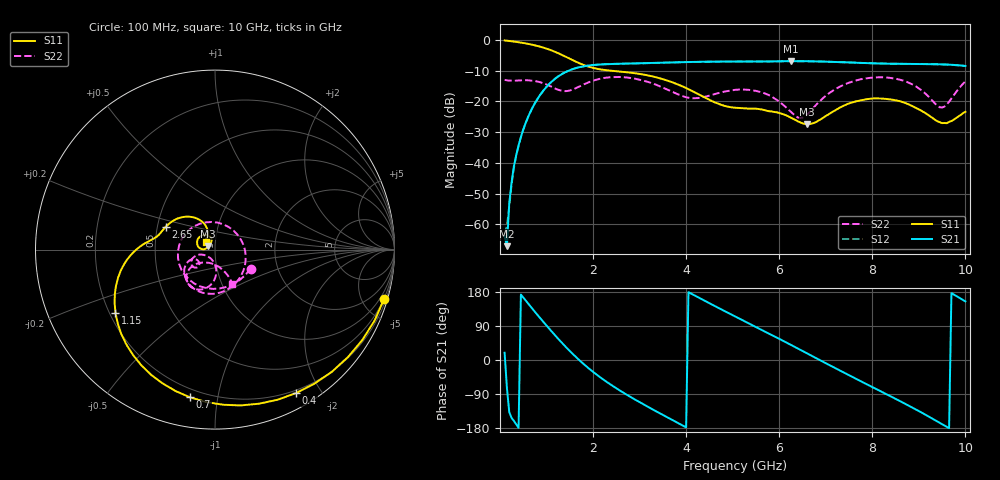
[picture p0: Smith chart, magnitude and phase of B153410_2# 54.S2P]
!  2-Port S-parameters saved by WinCal
! VAR MeasName=S-Parameters (CALIBRATED_DATA) read from VNA (N5245A)
! VAR MeasDate=2016-12-23 10:02:13
! VAR NAME=B153410_2# 54
! VAR FILENAME=B153410_2# 54.S2P
! VAR DATE=2016-12-23 10:02:13
! VAR PHYS_PORTS=1,2
# Hz S DB R 50
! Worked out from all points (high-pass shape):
!   199 points, 100 MHz to 10 GHz, reference 50 ohm
!   highest |S21| = -6.89 dB at 6.25 GHz (marker M1); lowest = -67.1 dB at 150 MHz (marker M2)
!   |S21| within 3 dB of the highest: 1.491 GHz to end of sweep
!   lowest |S11| = -27.4 dB at 6.6 GHz (marker M3), VSWR 1.09, Z = 46.3 + j1.88 ohm
!   |S11| at or under -10 dB: 2.386 GHz to end of sweep
!   |S22| runs from -25.4 to -12.0 dB; largest |S21 - S12| = 0.0019
!   S11 on the Smith chart (normalised r, x): 100 MHz: 0.46, -7.02; 400 MHz: 0.17, -1.70; 700 MHz: 0.15, -0.83; 1.15 GHz: 0.22, -0.28; 2.65 GHz: 0.55, +0.15; 10 GHz: 0.90, +0.08
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1e8  -0.16 -16.2  -63.69 19.3  -63.06 34.0  -12.97 -28.1
1.5e8  -0.24 -23.9  -67.07 -74.4  -60.59 -79.3  -13.12 -39.8
2e8  -0.33 -31.5  -53.02 -137.7  -54.10 -133.6  -13.22 -51.0
2.5e8  -0.42 -38.9  -46.35 -152.7  -46.99 -147.7  -13.22 -62.1
4e8  -0.74 -60.5  -34.27 -178.9  -34.47 -179.1  -13.18 -92.7
7e8  -1.57 -99.6  -22.00 134.8  -21.97 135.0  -13.23 -148.7
1.15e9  -3.65 -147.5  -13.05 69.9  -13.01 69.8  -15.52 121.1
1.75e9  -7.85 176.3  -8.72 -5.4  -8.70 -5.5  -14.83 -20.2
2.2e9  -9.67 166.5  -7.94 -49.7  -7.93 -49.8  -12.46 -79.5
2.65e9  -10.38 155.3  -7.72 -86.2  -7.72 -86.2  -12.11 -116.8
3.4e9  -12.32 130.7  -7.45 -138.4  -7.45 -138.5  -14.85 -153.1
4.2e9  -17.16 111.1  -7.13 169.2  -7.14 169.2  -18.95 -143.4
5.05e9  -22.04 126.0  -7.02 114.9  -7.04 115.0  -16.23 -140.5
5.7e9  -22.89 130.9  -7.00 74.4  -7.01 74.5  -17.44 -158.5
6.25e9  -25.30 132.6  -6.89 40.0  -6.92 39.9  -23.39 -153.7
6.6e9  -27.40 151.6  -6.91 17.4  -6.93 17.4  -24.26 -103.7
6.7e9  -27.23 159.9  -6.94 11.0  -6.96 10.9  -22.66 -94.3
7.4e9  -21.28 174.3  -7.26 -33.8  -7.26 -33.9  -14.49 -94.8
8.35e9  -19.27 135.8  -7.72 -93.1  -7.72 -93.0  -12.28 -127.0
8.9e9  -21.81 113.3  -7.81 -128.1  -7.82 -128.2  -14.79 -142.5
9.5e9  -27.04 121.6  -7.94 -169.3  -7.97 -169.3  -21.97 -102.8
1e10  -23.36 139.5  -8.44 154.7  -8.47 154.6  -13.45 -63.1
